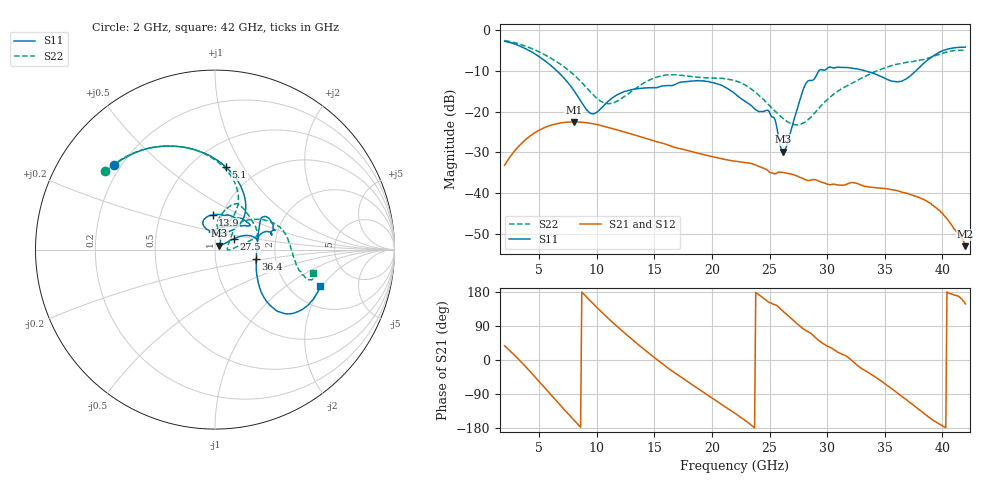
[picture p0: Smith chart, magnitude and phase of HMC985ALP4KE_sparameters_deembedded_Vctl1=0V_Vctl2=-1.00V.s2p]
!s2p File: Measurements: S11, S21, S12, S22
# GHz S dB R 50.0
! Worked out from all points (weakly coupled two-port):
!   401 points, 2 GHz to 42 GHz, reference 50 ohm
!   highest |S21| = -22.51 dB at 8 GHz (marker M1); lowest = -53.1 dB at 42 GHz (marker M2)
!   lowest |S11| = -29.8 dB at 26.2 GHz (marker M3), VSWR 1.07, Z = 52.4 + j2.27 ohm
!   |S11| at or under -10 dB: 6.549 GHz to 29.27 GHz (22.72 GHz wide, 127 % of centre); 33.35 GHz to 37.69 GHz (4.345 GHz wide, 12.2 % of centre)
!   |S22| runs from -23.3 to -2.5 dB; largest |S21 - S12| = 0.00014
!   S11 on the Smith chart (normalised r, x): 2 GHz: 0.17, +0.35; 5.1 GHz: 0.72, +0.84; 13.9 GHz: 0.90, +0.36; 27.5 GHz: 1.22, +0.15; 36.4 GHz: 1.58, -0.17; 42 GHz: 2.90, -1.91
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2  -2.68 140.2  -33.17 37.4  -33.18 37.4  -2.50 144.5
3.5  -4.11 112.4  -27.73 -7.3  -27.73 -7.3  -3.60 120.1
5.1  -6.68 82.3  -24.41 -60.2  -24.42 -60.2  -5.46 95.6
8  -14.75 45.6  -22.51 -158.0  -22.52 -158.1  -10.92 63.3
8.7  -17.82 51.8  -22.60 179.4  -22.60 179.3  -12.87 61.2
9.7  -20.54 85.7  -22.99 148.1  -22.99 148.1  -15.90 65.0
11  -17.41 114.5  -23.87 109.7  -23.88 109.7  -18.04 80.1
13.9  -14.24 93.9  -26.26 33.3  -26.27 33.3  -13.29 77.1
15.4  -13.94 73.0  -27.52 -2.6  -27.53 -2.6  -11.35 68.3
19.4  -12.52 34.6  -30.65 -88.0  -30.66 -88.0  -11.68 36.1
22  -15.61 52.3  -32.17 -140.6  -32.17 -140.6  -12.40 17.3
25  -20.19 97.9  -34.88 151.4  -34.89 151.4  -18.55 6.8
26.2  -29.80 41.9  -34.97 127.7  -35.00 127.6  -21.74 -0.9
27.5  -18.40 29.7  -35.98 92.8  -35.96 92.6  -23.18 5.3
28.1  -13.36 20.7  -36.73 78.7  -36.74 78.6  -22.52 16.5
28.7  -12.31 12.9  -36.71 67.4  -36.73 67.4  -21.00 27.6
31  -9.08 23.4  -38.04 19.7  -38.11 19.7  -14.82 48.1
33.3  -9.96 34.4  -38.39 -27.8  -38.38 -27.9  -11.35 38.3
35.4  -12.27 12.3  -39.09 -71.4  -39.09 -71.3  -8.89 23.9
36.4  -12.57 -12.8  -39.68 -94.0  -39.69 -94.0  -8.11 16.1
39.5  -5.80 -43.3  -43.71 -164.8  -43.81 -164.8  -6.12 -14.6
42  -4.14 -19.0  -53.07 147.9  -52.97 148.4  -5.00 -13.4
